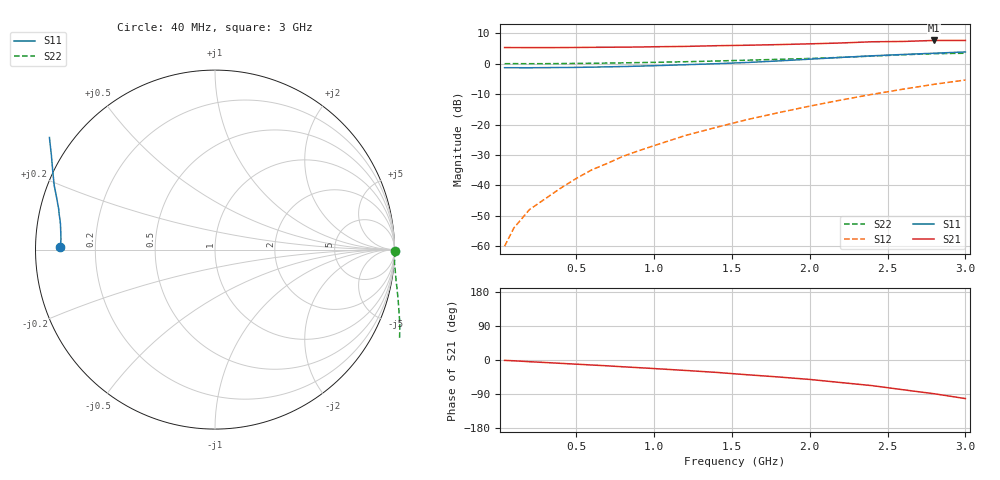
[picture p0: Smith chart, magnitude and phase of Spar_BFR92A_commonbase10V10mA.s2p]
! Filename:  BFR92ACH.S2P  Version:  2.0
! NXP part #: BFR92A  Date: Jul 1990
! Bias condition: Vce=10V, Ic=10mA
! COMMON BASE
#  MHz  S  MA  R  50
! Freq  S11  S21  S12  S22
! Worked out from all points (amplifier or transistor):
!   21 points, 40 MHz to 3 GHz, reference 50 ohm
!   highest |S21| = 7.7 dB at 2.8 GHz (marker M1)
!   |S21| within 3 dB of that: start of sweep to end of sweep
!   unconditionally stable (mu >= 1): nowhere
!   at 300 MHz: K = -0.54, MSG = 24.9 dB, |S12| = -44.4 dB
!   at 1 GHz: K = -0.94, MSG = 16.3 dB, |S12| = -26.9 dB
!   at 3 GHz: K = -0.87, MSG = 6.5 dB, |S12| = -5.4 dB
40  0.861 179.1  1.848 -1.0  0.001 56.0  1.002 -0.6
100  0.861 178.0  1.846 -2.1  0.002 84.0  1.004 -1.3
200  0.86 176.1  1.844 -4.5  0.004 104.9  1.002 -2.9
300  0.863 174.4  1.842 -6.6  0.006 120.2  1.003 -4.4
400  0.867 172.6  1.847 -8.8  0.009 127.8  1.008 -5.8
500  0.872 170.8  1.853 -11.0  0.013 132.7  1.013 -7.2
600  0.88 169.0  1.863 -13.2  0.018 136.9  1.019 -8.7
700  0.89 167.3  1.869 -15.4  0.023 140.0  1.026 -10.2
800  0.9 165.4  1.877 -17.9  0.03 141.9  1.035 -11.7
900  0.914 163.6  1.884 -20.2  0.037 143.5  1.045 -13.4
1000  0.929 161.8  1.904 -22.6  0.045 145.0  1.055 -14.9
1200  0.964 158.3  1.929 -27.5  0.066 145.8  1.08 -18.4
1400  1.002 154.4  1.981 -32.7  0.09 145.1  1.111 -22.0
1600  1.05 150.2  2.017 -39.0  0.121 144.6  1.145 -26.1
1800  1.114 145.9  2.066 -44.8  0.157 142.6  1.182 -30.8
2000  1.19 141.5  2.126 -51.3  0.201 139.8  1.221 -36.3
2200  1.272 136.9  2.196 -59.5  0.253 136.6  1.273 -42.8
2400  1.351 131.7  2.299 -67.6  0.314 132.2  1.338 -50.0
2600  1.421 125.0  2.328 -78.5  0.382 127.4  1.406 -57.9
2800  1.491 116.4  2.417 -89.1  0.46 120.8  1.464 -66.1
3000  1.564 107.3  2.417 -101.8  0.54 114.1  1.49 -75.5
